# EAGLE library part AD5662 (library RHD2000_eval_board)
Analog Devices AD5662 16-bit DAC
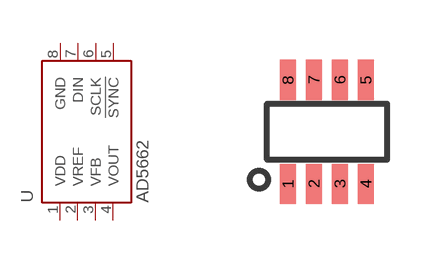
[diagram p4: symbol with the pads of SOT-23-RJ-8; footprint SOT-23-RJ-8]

Designator prefix U

## AD5662-SOT-23  [SOT-23-RJ-8]
1  VDD  pwr
2  VREF  in
3  VFB  pas
4  VOUT  out
5  !SYNC!  in
6  SCLK  in
7  DIN  in
8  GND  pwr

## Footprint SOT-23-RJ-8 (pad centres in mm)
smd 0.4 x 1: 1 -0.975,-1.3; 2 -0.325,-1.3; 3 0.325,-1.3; 4 0.975,-1.3; 5 0.975,1.3; 6 0.325,1.3; 7 -0.325,1.3; 8 -0.975,1.3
